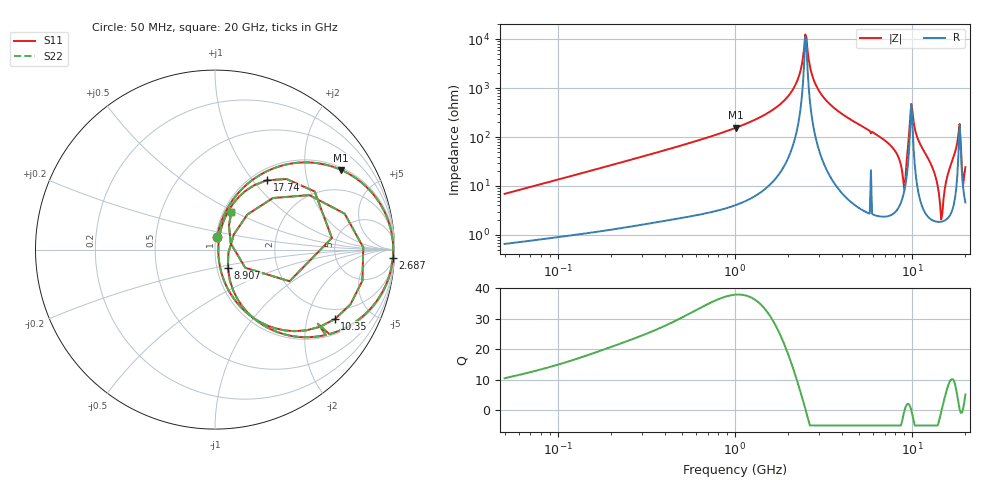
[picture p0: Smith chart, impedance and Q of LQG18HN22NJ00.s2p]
!Murata Part Number: LQG18HN22NJ00
!These Parameters are Measured in Series Mode Connection
!  o--[Z]--o
!Port1  Port2
!  o-------o
!Freq. Start=50[MHz] Stop=20[GHz], 401[Steps]
# Hz S RI R 50
!Freq.(Hz) S11(Real) S11(Imag) S21(Real) S21(Imag) S12(Real) S12(Imag) S22(Real) S22(Imag)
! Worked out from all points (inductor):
!   401 points, 50 MHz to 20 GHz, reference 50 ohm
!   read as one part in series: L = 21.7 nH near 51.52 MHz
!   highest Q = 37.9 at 1.015 GHz (marker M1), where L = 24.4 nH
!   self-resonance near 2.494 GHz
!   S11 on the Smith chart (normalised r, x): 50 MHz: 1.01, +0.14; 2.687 GHz: 8, -44; 8.907 GHz: 1.13, -0.24; 10.35 GHz: 1.55, -2.98; 17.74 GHz: 1.17, +1.18; 20 GHz: 1.09, +0.48
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5e7  0.0111 0.0676  0.9889 -0.0676  0.9889 -0.0676  0.0111 0.0676
1.364002e8  0.0416 0.1731  0.9584 -0.1731  0.9584 -0.1731  0.0416 0.1731
3.721004e8  0.2066 0.3867  0.7934 -0.3867  0.7934 -0.3867  0.2066 0.3867
1e9  0.6943 0.4477  0.3057 -0.4477  0.3057 -0.4477  0.6943 0.4477
1.015091e9  0.7027 0.4441  0.2973 -0.4441  0.2973 -0.4441  0.7027 0.4441
1.962148e9  0.9684 0.1512  0.0316 -0.1512  0.0316 -0.1512  0.9684 0.1512
2.279204e9  0.989 0.0602  0.011 -0.0602  0.011 -0.0602  0.989 0.0602
2.493527e9  0.9929 0.00367  0.00709 -0.00367  0.00709 -0.00367  0.9929 0.00367
2.687447e9  0.9911 -0.0442  0.00894 0.0442  0.00894 0.0442  0.9911 -0.0442
2.728004e9  0.9901 -0.0538  0.00988 0.0538  0.00988 0.0538  0.9901 -0.0538
3.680849e9  0.9278 -0.2451  0.0722 0.2451  0.0722 0.2451  0.9278 -0.2451
7.442007e9  0.3402 -0.4567  0.6598 0.4567  0.6598 0.4567  0.3402 -0.4567
8.264682e9  0.1742 -0.3425  0.8258 0.3425  0.8258 0.3425  0.1742 -0.3425
8.907419e9  0.0716 -0.1037  0.9284 0.1037  0.9284 0.1037  0.0716 -0.1037
9.600142e9  0.5255 0.3037  0.4745 -0.3037  0.4745 -0.3037  0.5255 0.3037
1.034674e10  0.6679 -0.387  0.3321 0.387  0.3321 0.387  0.6679 -0.387
1.295331e10  0.0746 -0.2252  0.9254 0.2252  0.9254 0.2252  0.0746 -0.2252
1.460232e10  0.0184 -0.00884  0.9816 0.00884  0.9816 0.00884  0.0184 -0.00884
1.774144e10  0.2899 0.3863  0.7101 -0.3863  0.7101 -0.3863  0.2899 0.3863
1.828096e10  0.5551 0.3239  0.4449 -0.3239  0.4449 -0.3239  0.5551 0.3239
1.912117e10  0.1689 -0.1014  0.8311 0.1014  0.8311 0.1014  0.1689 -0.1014
2e10  0.091 0.2067  0.909 -0.2067  0.909 -0.2067  0.091 0.2067
